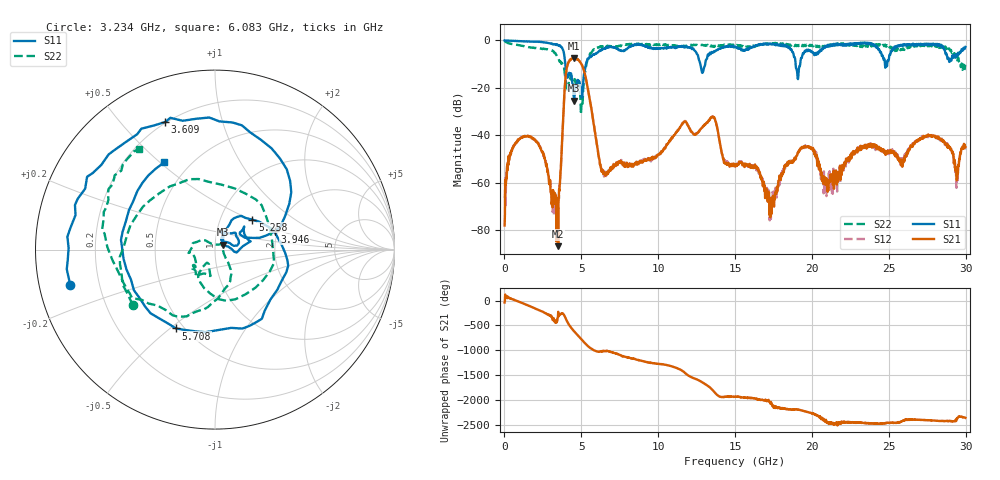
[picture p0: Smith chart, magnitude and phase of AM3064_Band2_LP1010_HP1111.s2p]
# Hz S DB R 50.0
!freq dBS11 angS11 dBS21 angS21 dBS12 angS12 dBS22 angS22
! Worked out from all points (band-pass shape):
!   1600 points, 10 MHz to 29.98 GHz, reference 50 ohm
!   highest |S21| = -7.35 dB at 4.508 GHz (marker M1); lowest = -86.8 dB at 3.496 GHz (marker M2)
!   |S21| within 3 dB of the highest: 4.101 GHz to 5.035 GHz (933.3 MHz wide, 20.4 % of centre)
!   lowest |S11| = -25.4 dB at 4.527 GHz (marker M3), VSWR 1.11, Z = 54.7 + j3.02 ohm
!   |S11| at or under -10 dB: 3.957 GHz to 5.302 GHz (1.344 GHz wide, 29 % of centre); 12.74 GHz to 13.06 GHz (318.8 MHz wide, 2.47 % of centre); 18.94 GHz to 19.23 GHz (296.7 MHz wide, 1.55 % of centre)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
!   |S22| runs from -31.2 to -0.3 dB; largest |S21 - S12| = 0.012
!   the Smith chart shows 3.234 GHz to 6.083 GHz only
!   S11 on the Smith chart (normalised r, x): 3.234 GHz: 0.09, -0.12; 3.609 GHz: 0.20, +0.66; 3.946 GHz: 1.93, +0.44; 5.258 GHz: 1.42, +0.51; 5.708 GHz: 0.45, -0.52; 6.083 GHz: 0.36, +0.52
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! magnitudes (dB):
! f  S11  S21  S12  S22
! 10 MHz  0.0  -78.0  -65.8  -0.3
! 366.1 MHz  -0.1  -48.7  -48.4  -1.3
! 1.378 GHz  -0.5  -40.4  -40.3  -2.6
! 3.234 GHz  -1.6  -67.0  -66.3  -5.2
! 3.496 GHz  -2.0  -86.8  -67.7  -7.5
! 3.609 GHz  -2.3  -60.3  -60.2  -9.0
! 3.946 GHz  -9.2  -17.6  -17.7  -14.9
! 4.508 GHz  -24.3  -7.4  -7.3  -16.9
! 4.527 GHz  -25.4  -7.4  -7.3  -16.8
! 5.015 GHz  -23.7  -10.0  -10.0  -26.4
! 5.258 GHz  -11.5  -15.0  -15.0  -12.9
! 5.708 GHz  -6.2  -31.1  -31.0  -4.6
! 6.083 GHz  -5.0  -46.7  -47.0  -3.1
! 10 GHz  -3.4  -48.1  -48.0  -1.8
! 13.54 GHz  -5.3  -32.2  -32.0  -2.6
! 15 GHz  -2.6  -53.2  -52.0  -1.8
! 17.39 GHz  -1.5  -68.9  -69.9  -1.3
! 19.99 GHz  -4.6  -45.9  -45.8  -1.9
! 20.89 GHz  -2.4  -58.3  -61.1  -2.7
! 25 GHz  -8.2  -46.7  -47.0  -2.3
! 29.4 GHz  -6.2  -58.5  -62.2  -6.8
! 29.98 GHz  -2.8  -45.0  -46.0  -10.2
